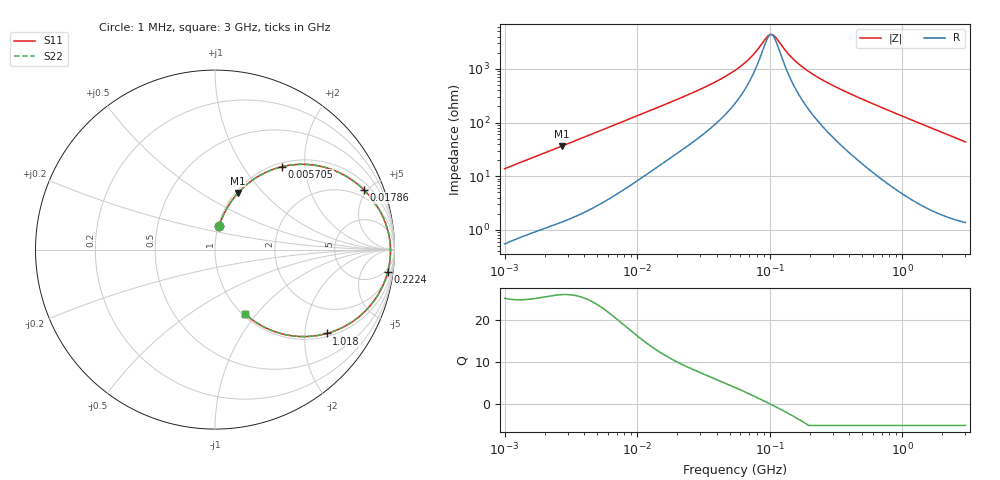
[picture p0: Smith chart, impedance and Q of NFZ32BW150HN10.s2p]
! NFZ32BW150HN10
# Hz S RI R 50
!Freq.(Hz) S11(Real) S11(Imag) S21(Real) S21(Imag) S12(Real) S12(Imag) S22(Real) S22(Imag)
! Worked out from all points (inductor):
!   401 points, 1 MHz to 3 GHz, reference 50 ohm
!   read as one part in series: L = 2.18 uH near 1.041 MHz
!   highest Q = 26.1 at 2.72 MHz (marker M1), where L = 2.14 uH
!   self-resonance near 102.4 MHz
!   S11 on the Smith chart (normalised r, x): 1 MHz: 1.01, +0.28; 5.705 MHz: 1.07, +1.53; 17.86 MHz: 1.44, +4.77; 222.4 MHz: 3, -15; 1.018 GHz: 1.09, -2.59; 3 GHz: 1.03, -0.87
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1000000  0.0238 0.1339  0.9762 -0.1339  0.9762 -0.1339  0.0238 0.1339
1751453  0.0615 0.2212  0.9385 -0.2212  0.9385 -0.2212  0.0615 0.2212
2720446  0.1277 0.3151  0.8723 -0.3151  0.8723 -0.3151  0.1277 0.3151
3823119  0.2173 0.3933  0.7827 -0.3933  0.7827 -0.3933  0.2173 0.3933
5705239  0.3736 0.462  0.6264 -0.462  0.6264 -0.462  0.3736 0.462
8861669  0.5791 0.4661  0.4209 -0.4661  0.4209 -0.4661  0.5791 0.4661
1.461624e7  0.7748 0.3797  0.2252 -0.3797  0.2252 -0.3797  0.7748 0.3797
1.785516e7  0.8302 0.3324  0.1698 -0.3324  0.1698 -0.3324  0.8302 0.3324
3.456417e7  0.9355 0.1823  0.0645 -0.1823  0.0645 -0.1823  0.9355 0.1823
5.477226e7  0.9652 0.0972  0.0348 -0.0972  0.0348 -0.0972  0.9652 0.0972
7.248696e7  0.9737 0.0522  0.0263 -0.0522  0.0263 -0.0522  0.9737 0.0522
9.593103e7  0.9774 0.0098  0.0226 -0.0098  0.0226 -0.0098  0.9774 0.0098
1.039275e8  0.9777 -0.00215  0.0223 0.00215  0.0223 0.00215  0.9777 -0.00215
1.103592e8  0.9777 -0.0111  0.0223 0.0111  0.0223 0.0111  0.9777 -0.0111
1.520175e8  0.9746 -0.0604  0.0254 0.0604  0.0254 0.0604  0.9746 -0.0604
2.094008e8  0.9648 -0.1149  0.0352 0.1149  0.0352 0.1149  0.9648 -0.1149
2.223601e8  0.962 -0.126  0.038 0.126  0.038 0.126  0.962 -0.126
4.480278e8  0.8884 -0.2821  0.1116 0.2821  0.1116 0.2821  0.8884 -0.2821
8.005644e8  0.7253 -0.4261  0.2747 0.4261  0.2747 0.4261  0.7253 -0.4261
1.017911e9  0.6229 -0.4673  0.3771 0.4673  0.3771 0.4673  0.6229 -0.4673
1.645649e9  0.3918 -0.4738  0.6082 0.4738  0.6082 0.4738  0.3918 -0.4738
3e9  0.1676 -0.3581  0.8324 0.3581  0.8324 0.3581  0.1676 -0.3581
